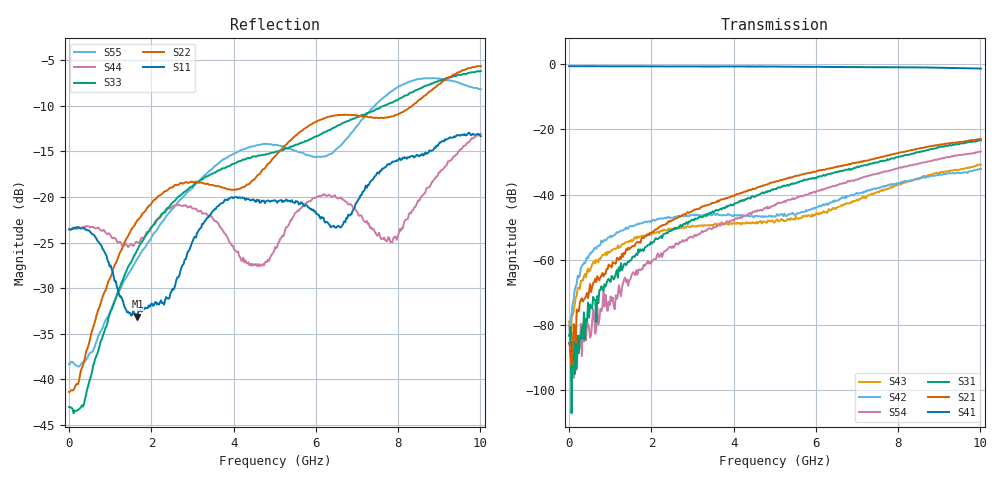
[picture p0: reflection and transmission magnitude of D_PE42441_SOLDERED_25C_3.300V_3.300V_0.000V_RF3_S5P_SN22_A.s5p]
! Device ID: PE42441
! Serial: 22
! Insertion: A
! Temp: 25C
! VDD: 3.300
! Control_Hi: 100.000
! Control_Lo: 0.000
! Logic State: RF3
! Port 1: RFC
! Port 2: RF1
! Port 3: RF2
! Port 4: RF3
! Port 5: RF4
! V1 = 0.00
! V2 = 3.30
! V3 = 0.00
! V4 = 0.00
! IDD: 1.083284e-04
! 1 Hz data is simulated
#  Hz  S  RI  R  50
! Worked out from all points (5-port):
!   402 points, 1 Hz to 10.01 GHz, reference 50 ohm
!   strongest paths, dB at 1 Hz, 2.485 GHz, 5.01 GHz, 7.51 GHz, 10.01 GHz:
!     S41: -0.7, -0.8, -0.8, -1.0, -1.4
!     S21: -85.5, -48.0, -36.1, -28.8, -23.0
!     S31: -83.2, -51.0, -38.3, -30.1, -23.4
!     S54: -80.0, -56.3, -43.3, -33.5, -26.8
!     S42: -85.8, -47.1, -46.8, -37.9, -32.1
!     S43: -78.9, -50.5, -48.1, -39.1, -30.9
!   lowest |S11| = -33.1 dB at 1.66 GHz (marker M1), VSWR 1.05, Z = 49.1 - j1.99 ohm
!   |S11| at or under -10 dB: start of sweep to end of sweep
